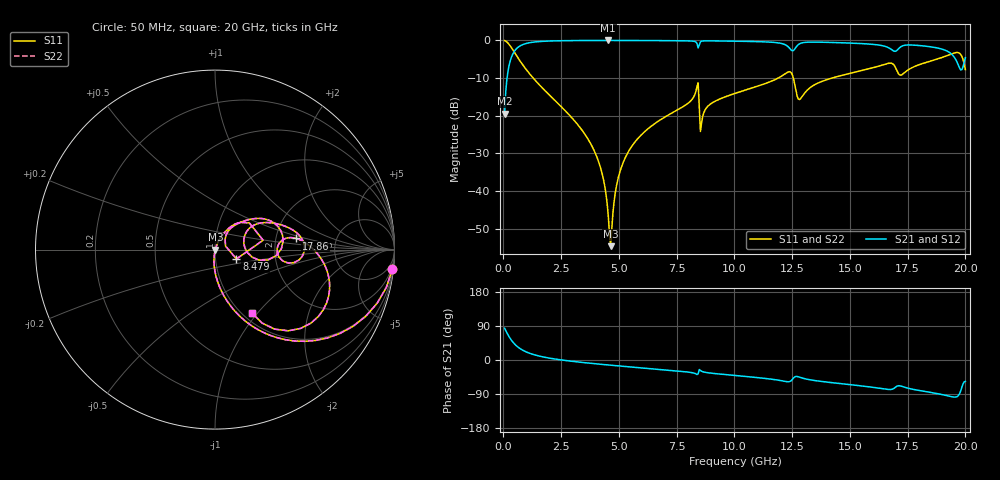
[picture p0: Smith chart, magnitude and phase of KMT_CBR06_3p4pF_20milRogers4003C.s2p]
! Data measured by Modelithics Inc. support@modelithics.com 813-866-6335
! KEMET CBR0603 3.4pF, Pad Width= 0.851mm, Pad Length= 0.64mm, Pad Gap= 0.62mm, 20mil Rogers 4003C substrate Data, January 2022
# hz S ma R 50
! 2 Port Network Data from SP1.SP block
! freq  magS11  angS11  magS21  angS21  magS12  angS12  magS22  angS22
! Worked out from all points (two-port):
!   401 points, 50 MHz to 20 GHz, reference 50 ohm
!   highest |S21| = -0.02 dB at 4.539 GHz (marker M1); lowest = -19.4 dB at 50 MHz (marker M2)
!   |S21| within 3 dB of the highest: 460.7 MHz to 19.26 GHz (18.8 GHz wide, 191 % of centre)
!   lowest |S11| = -54.6 dB at 4.638 GHz (marker M3), VSWR 1.00, Z = 50.2 - j0.022 ohm
!   |S11| at or under -10 dB: 1.289 GHz to 11.89 GHz (10.6 GHz wide, 161 % of centre); 12.55 GHz to 14.22 GHz (1.673 GHz wide, 12.5 % of centre)
!   |S22| runs from -54.6 to -0.1 dB; largest |S21 - S12| = 0
!   S11 on the Smith chart (normalised r, x): 50 MHz: 1, -18; 8.479 GHz: 1.26, -0.13; 17.86 GHz: 2.62, +0.41; 20 GHz: 1.10, -0.94
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5e7  0.9942 -6.3  0.1071 83.7  0.1071 83.7  0.9942 -6.3
2.99375e8  0.8391 -33.8  0.5432 56.2  0.5432 56.2  0.8391 -33.8
6.485e8  0.5745 -56.8  0.8176 33.1  0.8176 33.1  0.5745 -56.8
1.4465e9  0.2792 -77.8  0.9591 11.9  0.9591 11.9  0.2792 -77.8
3.391625e9  0.06503 -94.9  0.9962 -6.3  0.9962 -6.3  0.06503 -94.9
4.189625e9  0.02109 -96.4  0.9979 -11.2  0.9979 -11.2  0.02109 -96.4
4.53875e9  0.004709 -80.3  0.998 -13.2  0.998 -13.2  0.004709 -80.3
4.6385e9  0.001861 -6.8  0.998 -13.7  0.998 -13.7  0.001861 -6.8
4.93775e9  0.01362 66.6  0.9978 -15.4  0.9978 -15.4  0.01362 66.6
5.237e9  0.02628 68.7  0.9975 -17.0  0.9975 -17.0  0.02628 68.7
6.73325e9  0.08592 63.7  0.9937 -24.8  0.9937 -24.8  0.08592 63.7
8.32925e9  0.2085 46.8  0.9534 -36.4  0.9534 -36.4  0.2085 46.8
8.478875e9  0.1304 -23.5  0.8693 -25.1  0.8693 -25.1  0.1304 -23.5
8.6285e9  0.0984 51.8  0.9826 -30.9  0.9826 -30.9  0.0984 51.8
1.0025e10  0.1979 48.1  0.9761 -40.8  0.9761 -40.8  0.1979 48.1
1.231925e10  0.3803 16.8  0.827 -57.4  0.827 -57.4  0.3803 16.8
1.2818e10  0.1643 11.6  0.9004 -45.3  0.9004 -45.3  0.1643 11.6
1.336662e10  0.2466 32.3  0.9493 -53.2  0.9493 -53.2  0.2466 32.3
1.670825e10  0.4981 2.8  0.7895 -77.9  0.7895 -77.9  0.4981 2.8
1.785538e10  0.458 7.8  0.8619 -78.9  0.8619 -78.9  0.458 7.8
1.950125e10  0.6776 -19.7  0.6081 -97.8  0.6081 -97.8  0.6776 -19.7
2e10  0.4092 -59.6  0.5904 -56.3  0.5904 -56.3  0.4092 -59.6
